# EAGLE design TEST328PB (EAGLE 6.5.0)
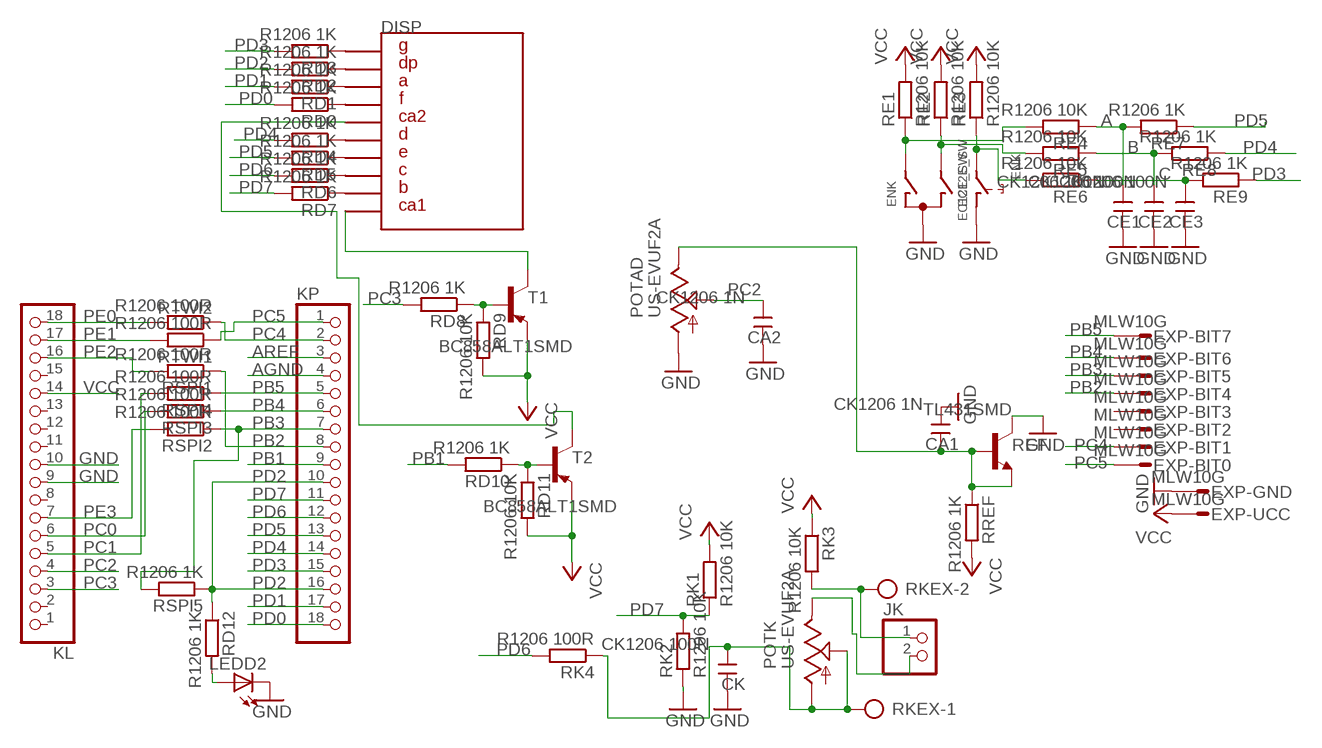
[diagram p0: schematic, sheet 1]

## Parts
CA1  CK1206 1N  CK+  [CK+]
CA2  CK1206 1N  CK+  [CK+]
CE1  CK1206 100N  CK+  [CK+]
CE2  CK1206 100N  CK+  [CK+]
CE3  CK1206 100N  CK+  [CK+]
CK  CK1206 100N  CK+  [CK+]
DISP  7SEG2SA7.62MM  [7SEG2CA7.63MM]
ENK  EC12E_SW  [ALPS_EC12E_SW]
EXP  MLW10G  PSL10MLW10G  [MLW10G]
JK  PINHD-1X2  [1X02]
KL  PINHD-1X18  [1X18]
KP  PINHD-1X18  [1X18]
LEDD2  LED5MM  [LED5MM]
POTAD  US-EVUF2A  [EVUF]
POTK  US-EVUF2A  [EVUF]
RD0  R1206 1K  R-EU_R1206  [R1206]
RD1  R1206 1K  R-EU_R1206  [R1206]
RD2  R1206 1K  R-EU_R1206  [R1206]
RD3  R1206 1K  R-EU_R1206  [R1206]
RD4  R1206 1K  R-EU_R1206  [R1206]
RD5  R1206 1K  R-EU_R1206  [R1206]
RD6  R1206 1K  R-EU_R1206  [R1206]
RD7  R1206 1K  R-EU_R1206  [R1206]
RD8  R1206 1K  R-EU_R1206  [R1206]
RD9  R1206 10K  R-EU_R1206  [R1206]
RD10  R1206 1K  R-EU_R1206  [R1206]
RD11  R1206 10K  R-EU_R1206  [R1206]
RD12  R1206 1K  R-EU_R1206  [R1206]
RE1  R1206 10K  R-EU_R1206  [R1206]
RE2  R1206 10K  R-EU_R1206  [R1206]
RE3  R1206 10K  R-EU_R1206  [R1206]
RE4  R1206 10K  R-EU_R1206  [R1206]
RE5  R1206 10K  R-EU_R1206  [R1206]
RE6  R1206 10K  R-EU_R1206  [R1206]
RE7  R1206 1K  R-EU_R1206  [R1206]
RE8  R1206 1K  R-EU_R1206  [R1206]
RE9  R1206 1K  R-EU_R1206  [R1206]
REF  TL431SMD  BC846  [SOT23]
RK1  R1206 10K  R-EU_R1206  [R1206]
RK2  R1206 10K  R-EU_R1206  [R1206]
RK3  R1206 10K  R-EU_R1206  [R1206]
RK4  R1206 100R  R-EU_R1206  [R1206]
RKEX  AK500/2  [AK500/2]
RREF  R1206 1K  R-EU_R1206  [R1206]
RSPI1  R1206 100R  R-EU_R1206  [R1206]
RSPI2  R1206 100R  R-EU_R1206  [R1206]
RSPI3  R1206 100R  R-EU_R1206  [R1206]
RSPI4  R1206 100R  R-EU_R1206  [R1206]
RSPI5  R1206 1K  R-EU_R1206  [R1206]
RTWI1  R1206 100R  R-EU_R1206  [R1206]
RTWI2  R1206 100R  R-EU_R1206  [R1206]
T1  BC858ALT1SMD  [SOT23-BEC]
T2  BC858ALT1SMD  [SOT23-BEC]

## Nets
A: CE1.2 RE4.1 RE7.2
AGND: KP.4
AREF: KP.3
B: CE2.2 RE5.1 RE8.2
C: CE3.2 RE6.1 RE9.2
GND: CA1.2 CA2.1 CE1.1 CE2.1 CE3.1 CK.1 ENK.C ENK.D EXP.10 KL.9 KL.10 LEDD2.K(C) POTAD.1(A) REF.3(C) RK2.1
N$1: ENK.A RE1.1 RE4.2
N$2: ENK.B RE2.1 RE5.2
N$3: DISP.4 RD0.1
N$4: CA1.1 POTAD.3(E) REF.1(B) REF.2(E) RREF.1
N$5: ENK.E RE3.1 RE6.2
N$6: RD8.1 RD9.1 T1.B
N$7: DISP.5 T2.C
N$8: RD10.1 RD11.1 T2.B
N$9: DISP.9 RD7.1
N$10: DISP.8 RD6.1
N$11: DISP.7 RD5.1
N$12: DISP.6 RD4.1
N$13: JK.1 RK3.2 RKEX.2
N$14: DISP.1 RD3.1
N$15: DISP.2 RD2.1
N$16: DISP.3 RD1.1
N$17: JK.2 POTK.3(E)
N$18: LEDD2.A RD12.2
N$24: CK.2 POTK.1(A) POTK.2(S) RK4.1 RKEX.1
N$26: DISP.10 T1.C
PB1: KP.9 RD10.2
PB2: EXP.5 KP.8 RSPI1.1
PB3: EXP.4 KP.7 RSPI2.1 RSPI5.2
PB4: EXP.3 KP.6 RSPI3.1
PB5: EXP.2 KP.5 RSPI4.1
PC0: KL.6 RSPI3.2
PC1: KL.5 RSPI4.2
PC2: CA2.2 KL.4 POTAD.2(S)
PC3: KL.3 RD8.2
PC4: EXP.8 KP.2 RTWI2.1
PC5: EXP.9 KP.1 RTWI1.1
PD0: KP.18 RD0.2
PD1: KP.17 RD1.2
PD2: KP.10 KP.16 RD2.2 RD12.1 RSPI5.1
PD3: KP.15 RD3.2 RE9.1
PD4: KP.14 RD4.2 RE8.1
PD5: KP.13 RD5.2 RE7.1
PD6: KP.12 RD6.2 RK4.2
PD7: KP.11 RD7.2 RK1.1 RK2.2
PE0: KL.18 RTWI2.2
PE1: KL.17 RTWI1.2
PE2: KL.16 RSPI1.2
PE3: KL.7 RSPI2.2
VCC: EXP.1 KL.14 RD9.2 RD11.2 RE1.2 RE2.2 RE3.2 RK1.2 RK3.1 RREF.2 T1.E T2.E
Unconnected: ENK.GND1(G) ENK.GND2(G) EXP.6 EXP.7 KL.1 KL.2 KL.8 KL.11 KL.12 KL.13 KL.15

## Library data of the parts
CA1 CA2 CE1-CE3 CK = !MOJE:CK+
DISP = MATLIB:7SEG2SA7.62MM
ENK = switch-alps:EC12E_SW: ALPS rotary Encoder EC12E series with switch; MPN: EC12E2424407; OC_FARNELL: 1520813; OC_NEWARK: 74M1068
EXP = !MOJE:PSL10: CONNECTOR
JK = pinhead:PINHD-1X2: PIN HEADER
KL KP = pinhead:PINHD-1X18: PIN HEADER
LEDD2 = led:LED: LED
POTAD POTK = pot:US-EVU: 9 mm Square Rotary Potentiometers Source: Panasonic
RD0 RD1-RD12 RE1-RE9 RK1-RK4 RREF RSPI1-RSPI5 RTWI1 RTWI2 = rcl:R-EU_: RESISTOR, European symbol
REF = transistor:BC846: NPN TRANSISTOR
RKEX = con-ptr500:AK500/2: CONNECTOR; OC_FARNELL: unknown; OC_NEWARK: unknown
T1 T2 = transistor-pnp:BC858*: PNP Transistror

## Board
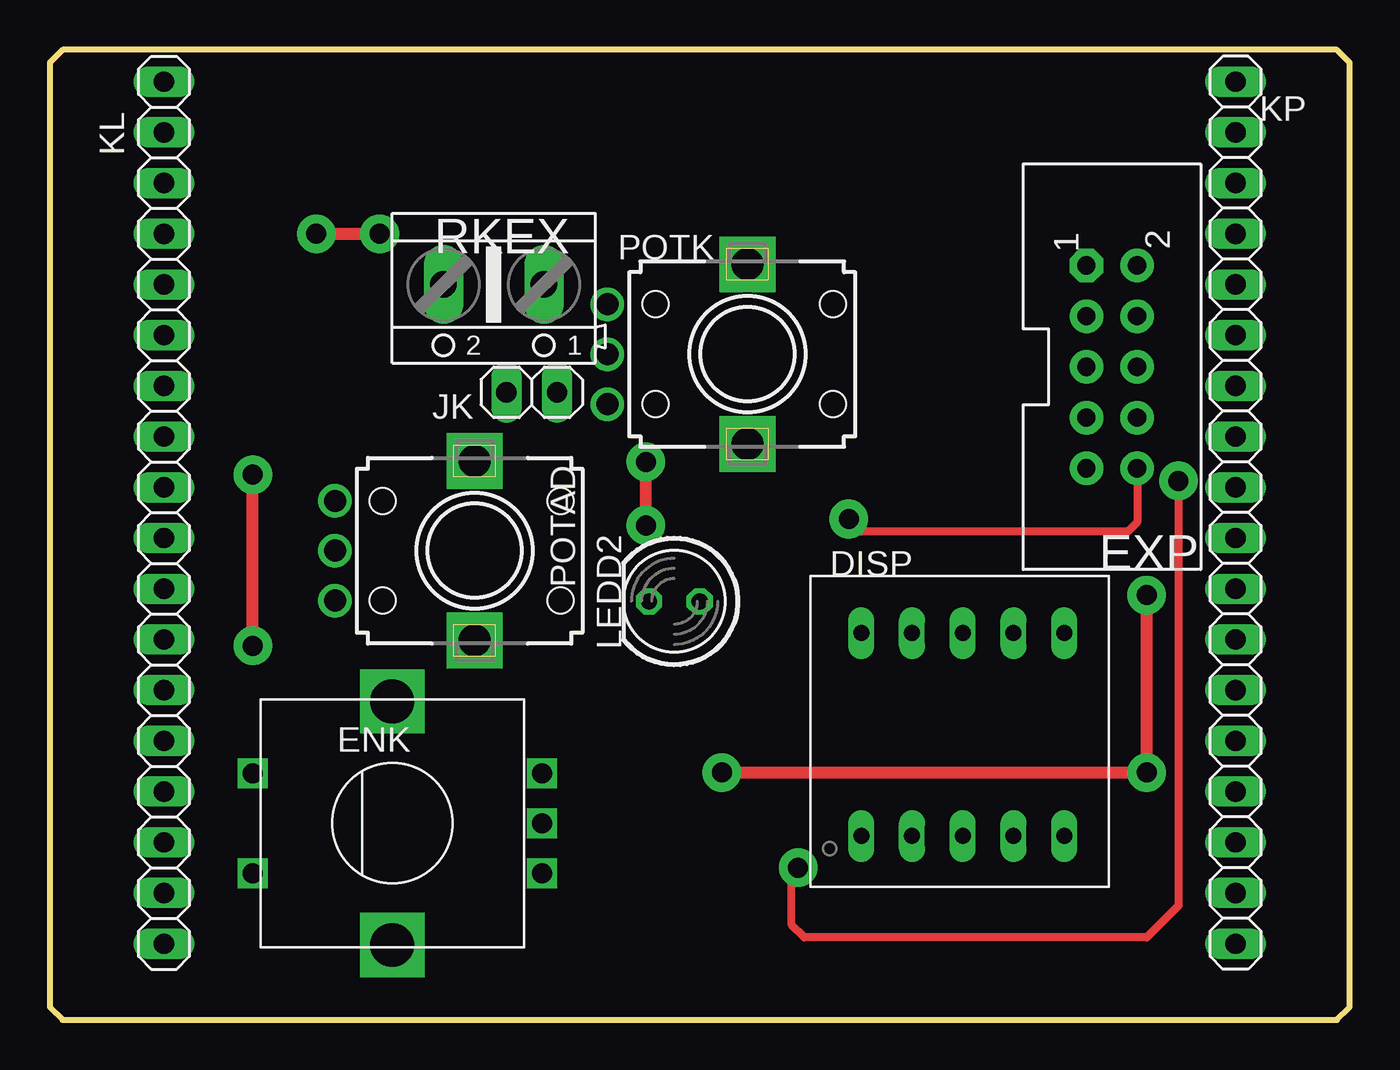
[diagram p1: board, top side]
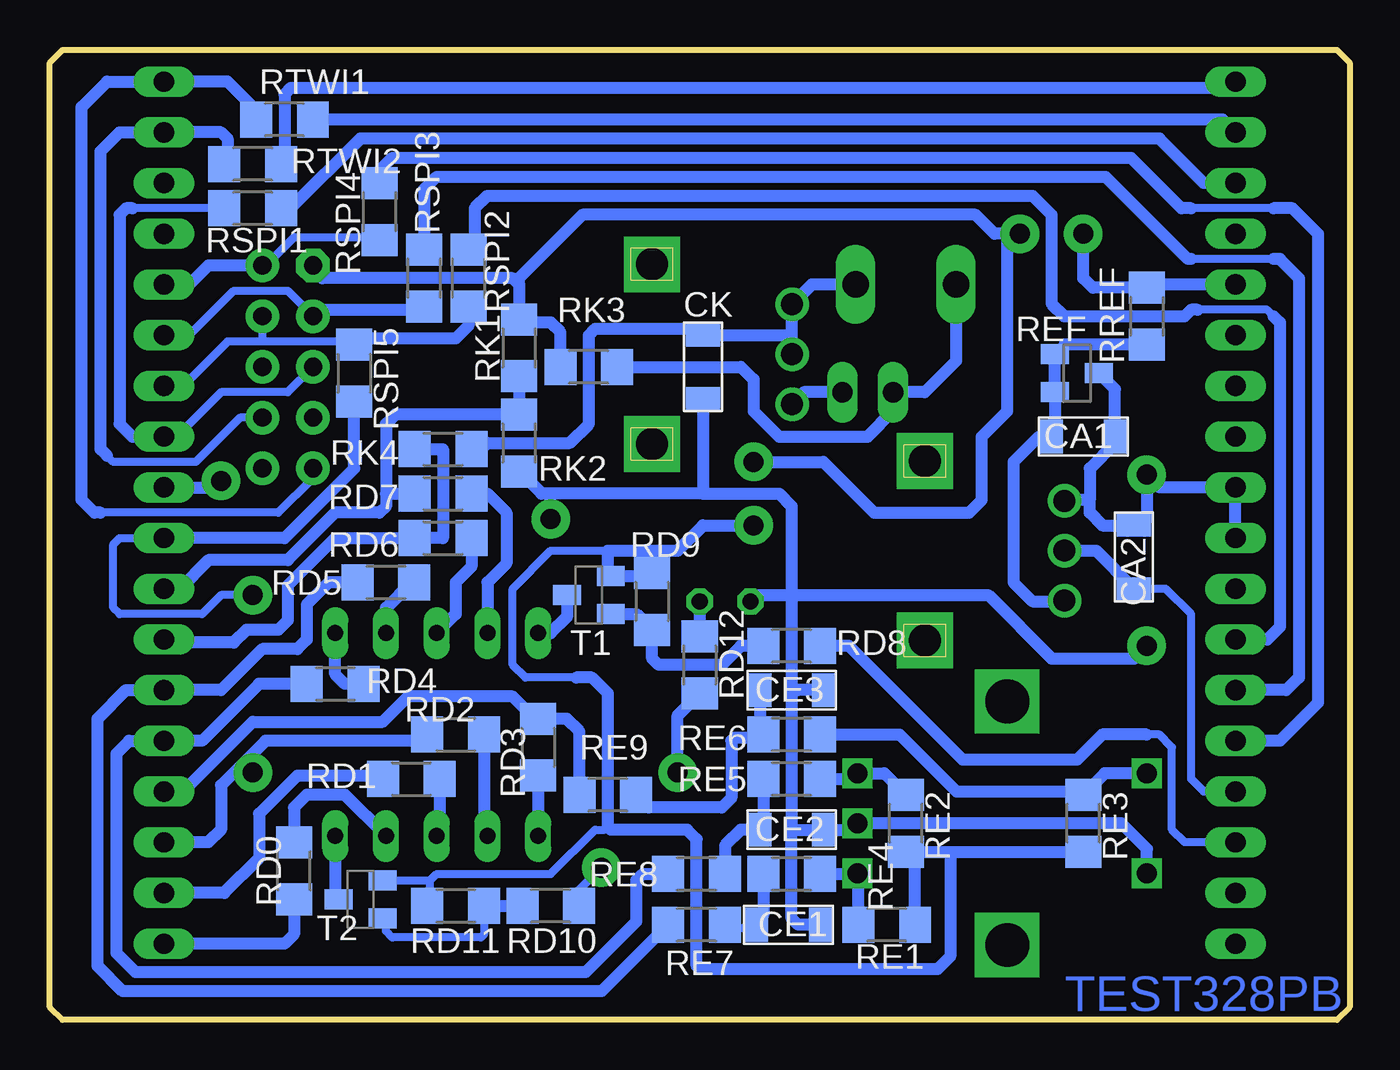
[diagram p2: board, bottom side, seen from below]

Size 65.09 x 48.58 mm. Coordinates in mm from the lower left corner, seen from the top.
Outline: 0,47.94 0,0.64 0.64,0 64.45,0 65.09,0.64 65.09,47.94 64.45,48.58 0.64,48.58 0,47.94
Copper layers (1*16): Top 0.035mm / dielectric 1.5mm / Bottom 0.035mm
Design rules "default": minimum track width 10mil, minimum drill 24mil, track to track 8mil, track to pad 8mil, pad to pad 8mil, via to via 8mil, smd to smd 8mil, copper to edge 40mil, drill to drill 8mil, minimum pad ring 10mil, minimum via ring 8mil, stop-mask expansion 4mil, vias tented up to drill 0mil, thermal gap 10mil

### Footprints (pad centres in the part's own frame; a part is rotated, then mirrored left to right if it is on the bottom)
CK+ = smd 1.14 x 1.7: 1 -1.587,0; 2 1.587,0
7SEG2CA7.63MM = drill 0.8 long: 1 -4.763,-4.763; 2 -2.223,-4.763; 3 0.318,-4.763; 4 2.857,-4.763; 5 5.397,-4.763; 6 5.397,5.397; 7 2.857,5.397; 8 0.318,5.397; 9 -2.223,5.397; 10 -4.763,5.397
ALPS_EC12E_SW = drill 1 square: A -2.5,-7.5; B 2.5,-7.5; C 0,-7.5; D -2.5,7; E 2.5,7 | drill 2.2 square: GND1 -6.1,0; GND2 6.1,0
MLW10G = drill 0.914 pad 1.676 octagon: 1 -5.08,-1.27 | drill 0.914 pad 1.676: 2 -5.08,1.27; 3 -2.54,-1.27; 4 -2.54,1.27; 5 0,-1.27; 6 0,1.27; 7 2.54,-1.27; 8 2.54,1.27; 9 5.08,-1.27; 10 5.08,1.27
1X02 = drill 1.016 long: 1 -1.27,0; 2 1.27,0
1X18 = drill 1.016 long: 1 -21.59,0; 2 -19.05,0; 3 -16.51,0; 4 -13.97,0; 5 -11.43,0; 6 -8.89,0; 7 -6.35,0; 8 -3.81,0; 9 -1.27,0; 10 1.27,0; 11 3.81,0; 12 6.35,0; 13 8.89,0; 14 11.43,0; 15 13.97,0; 16 16.51,0; 17 19.05,0; 18 21.59,0
LED5MM = drill 0.813 octagon: A -1.27,0; K 1.27,0
EVUF = drill 1.1 pad 1.676: 1 -2.5,-7; 2 0,-7; 3 2.5,-7 | drill 1.6 pad 2.8 square: M1 4.5,0; M2 -4.5,0
R1206 = smd 1.6 x 1.803: 1 -1.422,0; 2 1.422,0
SOT23 = smd 1 x 1.4: 1 -0.95,-1.1; 2 0.95,-1.1; 3 0,1.1
AK500/2 = drill 1.321 long: 1 -2.515,0; 2 2.515,0
SOT23-BEC = smd 1 x 1.4: B -0.95,-1.1; C 0,1.1; E 0.95,-1.1

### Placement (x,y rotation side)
CA1  13.34,29.21 0 bottom
CA2  10.79,23.18 270 bottom
CE1  28.1,4.76 180 bottom
CE2  27.94,9.53 180 bottom
CE3  27.94,16.51 180 bottom
CK  32.38,32.7 90 bottom
DISP  45.4,13.97 0 top
ENK  17.14,9.84 90 top
EXP  53.18,32.7 270 top
JK  24.13,31.43 0 top
KL  5.71,25.4 90 top
KP  59.37,25.4 270 top
LEDD2  31.27,20.95 180 top
POTAD  21.27,23.5 270 top
POTK  34.92,33.34 270 top
RD0  52.86,7.46 270 bottom
RD1  46.99,12.06 180 bottom
RD2  44.77,14.29 180 bottom
RD3  40.64,13.65 90 bottom
RD4  50.8,16.83 180 bottom
RD5  48.26,21.91 180 bottom
RD6  45.4,24.13 180 bottom
RD7  45.4,26.35 180 bottom
RD8  27.94,18.73 0 bottom
RD9  34.92,20.95 90 bottom
RD10  40.01,5.71 0 bottom
RD11  44.77,5.71 180 bottom
RD12  32.54,17.78 90 bottom
RE1  23.18,4.76 0 bottom
RE2  22.23,9.84 270 bottom
RE3  13.34,9.84 270 bottom
RE4  27.94,7.3 0 bottom
RE5  27.94,12.06 0 bottom
RE6  27.94,14.29 0 bottom
RE7  32.7,4.76 0 bottom
RE8  32.7,7.3 0 bottom
RE9  37.15,11.27 0 bottom
REF  13.65,32.38 270 bottom
RK1  41.59,33.66 90 bottom
RK2  41.59,28.89 90 bottom
RK3  38.1,32.7 0 bottom
RK4  45.4,28.57 180 bottom
RKEX  22.23,36.83 180 top
RREF  10.16,35.24 90 bottom
RSPI1  54.93,40.64 0 bottom
RSPI2  44.13,37.15 90 bottom
RSPI3  46.35,37.15 90 bottom
RSPI4  48.58,40.48 90 bottom
RSPI5  49.85,32.38 90 bottom
RTWI1  53.34,45.09 0 bottom
RTWI2  54.93,42.86 0 bottom
T1  38.1,21.27 90 bottom
T2  49.53,6.03 90 bottom

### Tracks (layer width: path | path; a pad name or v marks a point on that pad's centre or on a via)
A
  Bottom 0.406: RE7.2 31.27,4.6 30.64,4.6 30.01,4.6 CE1.2
  Bottom 0.61: RE4.1 29.36,5.25 CE1.2
B
  Bottom 0.406: 29.36,9.69 CE2.2 29.69,9.36
  Bottom 0.61: RE5.1 29.36,9.69 | CE2.2 30.48,9.53 31.27,8.73 RE8.2
C
  Bottom 0.406: 29.84,14.76 29.38,14.76 29.21,14.92 29.21,14.44 RE6.1
  Bottom 0.61: CE3.2 29.53,15.07 29.84,14.76 29.84,14.45 29.53,14.13 30.8,14.13 30.96,13.97 30.96,11.11 31.43,10.64 35.09,10.64 RE9.2
GND  (via drill 1 pad 1.93)
  Top 0.406: EXP.10 54.45,24.92 53.98,24.45 40.64,24.45 v40.01,25.08
  Top 0.61: v10.16,18.73 v10.16,27.3
  Bottom 0.406: 27.62,16.51 27.94,16.19 | 11.11,24.77 CA2.1 10.48,25.08 10.16,25.08
  Bottom 0.61: CE1.1 27.62,4.76 27.94,5.08 27.94,9.53 | 27.94,9.53 CE2.1 24.96,9.53 ENK.C 11.43,9.84 10.14,8.56 ENK.D | CE3.1 27.62,16.51 | 27.94,9.53 27.94,16.19 27.94,21.27 | REF.3 11.75,31.58 CA1.2 11.75,28.89 13.02,27.62 13.02,26.04 | CK.1 32.38,26.35 | 32.38,26.35 40.01,26.35 | 40.01,26.35 40.47,26.35 RK2.1 | 32.38,26.35 28.57,26.35 27.94,25.72 27.94,21.27 | 27.94,21.27 18.1,21.27 14.92,18.1 10.79,18.1 v10.16,18.73 | 10.16,25.08 v10.16,27.3 9.53,26.67 KL.10 KL.9 | v40.01,25.08 40.01,26.35 | CA2.1 12.38,24.77 13.02,25.4 13.02,26.04 | 13.02,26.04 14.23,26.04 POTAD.1 | LEDD2.K 29.69,21.27 27.94,21.27
N$1
  Bottom 0.406: 24.6,7.3 ENK.A 24.68,7.3
  Bottom 0.61: RE1.1 24.6,7.3 | RE4.2 24.68,7.3
N$2
  Bottom 0.61: RE5.2 24.92,12.06 ENK.B 23.3,12.34 RE2.1
N$3
  Bottom 0.61: DISP.4 50.32,11.27 52.23,11.27 52.86,10.64 RD0.1
N$4
  Bottom 0.406: REF.1 14.27,33.82 | 14.75,30.02 14.92,29.84 | CA1.1 15.56,29.21 | 14.31,20.95 POTAD.3
  Bottom 0.61: RREF.1 14.27,33.82 | REF.1 REF.2 14.75,30.02 | 14.92,29.84 CA1.1 | 15.56,29.21 16.83,27.94 16.83,21.91 15.88,20.95 14.31,20.95
N$5
  Bottom 0.406: 13.17,11.43 RE3.1
  Bottom 0.61: ENK.E 12.26,12.34 13.17,11.43 19.68,11.43 22.54,14.29 RE6.2
N$6
  Bottom 0.61: T1.B 35.72,20.32 RD9.1 34.92,18.1 34.61,17.78 31.43,17.78 30.48,18.73 RD8.1
N$7
  Bottom 0.406: 50.8,6.2 T2.C
  Bottom 0.61: DISP.5 50.8,6.2
N$8
  Bottom 0.406: RD11.1 43.35,4.28 43.5,4.13 47.94,4.13 48.26,4.45 48.26,4.91 T2.B
  Bottom 0.61: RD11.1 RD10.1
N$9
  Bottom 0.61: RD7.1 43.18,26.35 42.23,25.4 42.23,22.86 43.18,21.91 DISP.9
N$10
  Bottom 0.61: RD6.1 43.98,22.7 44.77,21.91 44.77,20.32 DISP.8
N$11
  Bottom 0.61: RD5.1 46.99,21.91 48.26,20.64 DISP.7
N$12
  Bottom 0.61: RD4.1 50.32,16.83 50.8,17.3 DISP.6
N$13
  Bottom 0.61: RKEX.2 19.71,32.99 21.27,31.43 JK.1 22.86,30.48 24.13,29.21 28.57,29.21 29.84,30.48 29.84,32.07 30.48,32.7 RK3.2
N$14
  Bottom 0.61: 40.81,9.37 DISP.1 RD3.1
N$15
  Bottom 0.61: RD2.1 43.35,9.37 DISP.2
N$16
  Bottom 0.61: RD1.1 45.57,9.36 DISP.3
N$17
  Bottom 0.61: JK.2 27.33,31.43 POTK.3
N$18
  Bottom 0.61: RD12.2 LEDD2.A
N$24
  Bottom 0.406: 43.81,28.89 43.5,28.57 RK4.1
  Bottom 0.61: 43.5,28.57 43.18,28.89 39.05,28.89 38.1,29.84 38.1,34.29 37.78,34.61 32.7,34.61 CK.2 27.94,34.29 27.94,33.35 POTK.2 POTK.1 26.93,36.83 RKEX.1
N$26
  Bottom 0.61: T1.C 39.2,20.17 40.01,19.37 DISP.10
PB1  (via drill 1 pad 1.93)
  Top 0.406: v56.52,26.99 56.52,5.71 54.93,4.13 37.78,4.13 37.15,4.76 37.15,7.3 v37.47,7.62
  Bottom 0.406: RD10.2 38.58,6.18 38.73,6.35 v37.47,7.62
  Bottom 0.61: KP.9 56.83,26.67 v56.52,26.99
PB2
  Bottom 0.406: EXP.5 53.18,31.43 56.52,31.43 58.42,29.53 59.05,29.53 KP.8 | RSPI1.1 60.96,40.64
  Bottom 0.61: KP.8 60.96,29.21 61.59,29.84 61.59,40.32 61.28,40.64 60.96,40.64
PB3
  Bottom 0.406: RSPI5.2 49.85,33.66 50.16,33.97 54.45,33.97 | 54.45,33.97 56.2,33.97 58.42,31.75 KP.7 | EXP.4 54.45,33.97
  Bottom 0.61: RSPI2.1 44.13,34.77 44.77,34.13 49.52,34.13 RSPI5.2
PB4
  Bottom 0.406: 46.52,35.56 RSPI3.1 | KP.6 58.1,34.29 55.88,36.51 53.18,36.51 EXP.3
  Bottom 0.61: 46.52,35.56 52.07,35.56 EXP.3
PB5
  Bottom 0.406: RSPI4.1 49.05,39.05 48.9,39.05 49.21,39.21 52.86,39.21 54.29,37.78 EXP.2
  Bottom 0.61: EXP.2 57.15,37.78 58.1,36.83 KP.5
PC0
  Bottom 0.406: 3.81,38.1 7.94,38.1
  Bottom 0.61: KL.6 3.17,16.51 2.54,17.14 2.54,37.15 3.49,38.1 3.81,38.1 | RSPI3.2 46.35,41.59 45.72,42.23 12.22,42.23 8.1,38.1 7.94,38.1
PC1
  Bottom 0.406: 3.81,40.64 7.94,40.64
  Bottom 0.61: KL.5 3.49,13.97 1.59,15.88 1.59,39.37 2.86,40.64 3.81,40.64 | RSPI4.2 48.58,42.55 47.94,43.18 10.95,43.18 8.41,40.64 7.94,40.64
PC2
  Bottom 0.406: KL.4 7.3,11.43 7.94,12.06 7.94,20.32 9.21,21.59 CA2.2
  Bottom 0.61: POTAD.2 12.7,23.5 CA2.2
PC3
  Bottom 0.406: KL.3 8.26,8.89 8.89,9.53 8.89,13.65 9.53,14.29 10.16,14.29
  Bottom 0.61: 10.16,14.29 12.38,14.29 13.65,13.02 19.37,13.02 25.08,18.73 RD8.2
PC4
  Bottom 0.406: 56.2,43.01 RTWI2.1 | EXP.8 55.56,30.16 57.78,27.94 61.91,27.94 62.23,28.26
  Bottom 0.61: 56.2,43.01 56.2,44.13 56.52,44.45 KP.2 61.59,44.45 62.55,43.5 62.55,28.57 62.23,28.26
PC5
  Bottom 0.406: RTWI1.1 54.76,45.55 | 62.55,25.4 53.66,25.4 51.91,27.15 EXP.9
  Bottom 0.61: 54.76,45.55 56.2,46.99 KP.1 62.23,46.99 63.5,45.72 63.5,26.04 62.87,25.4 62.55,25.4
PD0
  Bottom 0.61: RD0.2 52.86,4.29 53.34,3.81 KP.18
PD1
  Bottom 0.61: RD1.2 48.9,12.06 49.05,12.22 52.7,12.22 54.61,10.32 54.61,8.1 56.36,6.35 KP.17
PD2  (via drill 1 pad 1.93)
  Top 0.61: v54.93,21.27 v54.93,12.38 v33.66,12.38
  Bottom 0.406: 54.29,13.97 54.93,13.34 v54.93,12.38 | v54.93,21.27 56.52,21.27 57.47,20.32 61.59,20.32 61.91,20.64 61.91,23.81 61.59,24.13 KP.10
  Bottom 0.61: RD2.2 46.35,13.97 54.29,13.97 56.52,11.75 56.52,9.53 57.15,8.89 KP.16 | RSPI5.1 49.85,27.62 53.34,24.13 KP.10 | v33.66,12.38 33.66,15.25 RD12.1
PD3
  Bottom 0.406: RD3.2 40.79,15.07
  Bottom 0.61: KP.15 58.42,11.43 54.93,14.92 48.42,14.92 47.15,16.19 41.91,16.19 40.79,15.07 | RE9.1 38.57,14.44 39.21,15.08 RD3.2
PD4
  Bottom 0.61: RD4.2 54.61,16.83 57.47,13.97 KP.14 61.12,13.97 61.75,13.34 61.75,3.33 60.8,2.38 38.26,2.38 35.72,4.92 35.72,6.99 35.4,7.3 RE8.1
PD5
  Bottom 0.61: RD5.2 51.12,21.91 52.23,20.8 52.23,19.05 52.7,18.57 54.45,18.57 56.52,16.51 KP.13 61.28,16.51 62.71,15.08 62.71,2.7 61.44,1.43 37.46,1.43 RE7.1
PD6
  Bottom 0.61: RK4.2 45.4,28.57 45.4,24.13 RD6.2 50.8,24.13 53.18,21.75 53.18,20 53.66,19.53 55.24,19.53 55.88,18.89 59.21,18.89 KP.12
PD7
  Bottom 0.406: RK2.2 41.59,30.16 41.91,29.84 41.91,30 RK2.2
  Bottom 0.61: RK1.1 RK2.2 47.79,30.31 48.26,29.84 48.26,26.35 | 48.26,26.35 RD7.2 | 48.26,26.35 48.26,25.72 48.58,25.4 50.8,25.4 53.18,23.02 57.15,23.02 58.58,21.59 KP.11
PE0
  Bottom 0.61: KL.18 6.03,46.67 53.02,46.67 53.34,46.35 53.34,43.03 RTWI2.2
PE1
  Bottom 0.61: KL.17 6.35,45.09 RTWI1.2
PE2
  Bottom 0.406: 53.02,40.64 RSPI1.2
  Bottom 0.61: KL.16 7.3,41.91 9.53,44.13 49.53,44.13 53.02,40.64
PE3
  Bottom 0.406: 43.81,38.89 RSPI2.2 | 3.81,35.24 4.13,35.56 7.62,35.56
  Bottom 0.61: KL.7 4.13,19.05 3.49,19.68 3.49,34.92 3.81,35.24 | 43.81,38.89 43.81,40.64 43.18,41.27 15.88,41.27 14.92,40.32 14.92,35.88 14.29,35.24 8.26,35.24 7.94,35.56 7.62,35.56
VCC  (via drill 1 pad 1.93)
  Top 0.61: v13.34,39.37 v16.51,39.37 | v29.84,24.77 v29.84,27.94
  Bottom 0.406: 21.76,7.95 RE2.2 20.15,8.42 20,8.26 | 9.36,36.83 RREF.2 | T2.E 46.04,6.98 46.04,6.99 | 46.04,6.35 46.04,5.87 RD11.2 46.19,5.88 45.72,6.35 46.04,6.35 | 46.04,6.35 46.04,6.99 | 46.04,6.99 45.72,7.3 40.01,7.3 37.78,9.53 37.31,9.53 37.15,9.68 | 38.73,17.14 41.27,17.14 41.91,17.78 41.91,21.59 40.01,23.5 37.15,23.5 | 37.15,22.37 T1.E | 41.59,37.15 41.59,36.83
  Bottom 0.61: RE1.2 21.76,7.95 | RE2.2 RE3.2 | KL.14 9.36,36.83 | RREF.2 12.85,36.66 13.34,37.15 v13.34,39.37 | v16.51,39.37 17.14,39.37 | 17.14,39.37 17.78,39.37 18.73,40.32 38.42,40.32 41.59,37.15 | v29.84,24.77 32.38,24.77 33.66,23.5 37.15,23.5 37.15,22.37 | v29.84,27.94 26.35,27.94 23.81,25.4 19.05,25.4 18.41,26.04 18.41,29.21 17.14,30.48 17.14,39.37 | 20,8.26 20,3.17 20.64,2.54 32.54,2.54 32.7,2.7 32.7,9.05 33.18,9.53 36.99,9.53 37.15,9.68 37.15,16.35 37.94,17.14 38.73,17.14 | EXP.1 51.44,37.15 41.91,37.15 41.59,36.83 RK1.2 41.44,34.92 40.01,34.92 39.52,34.44 RK3.1 | T1.E 35.08,22.22 RD9.2

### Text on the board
Bottom: TEST328PB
